(* Logix 5000 AddOnInstructionDefinition export AMCI_SV160E2_Axis_Follower_Circular; software revision 20.03 *)

ADD_ON_INSTRUCTION AMCI_SV160E2_Axis_Follower_Circular   (* revision 1.0, vendor AMCI, ExecuteEnableInFalse *)
// Revision note:
// 8/2019 Version 0 Initial release of SV160E2 Add On Instructions.
// 3/17/20 Version 13/17/20 Version 1 replaced the generic EDS file with a more complete V1.6 EDS file.  Also added a line of code to limit the minimum follower acceleration to -15999.
// Help:
// 2/2017: V0 is the initial release
// 7/2017: V1 added enable and error bits.
// 5/2019: V2 added unlatching the error bit when the rung goes false and the ability to select between normal (jog CCW) and continuous follower (jog CW)
VAR_OUTPUT
   EN : BOOL; {visible}
END_VAR
VAR_INPUT
   Status_Word_0 : INT; {required}
        .0   // set when moving CW
        .1   // set when moving CCW
        .3   // set when stopped
   Status_Word_1 : INT; {required}
        .15   // 0 when disabled 1 when enabled
   Follower_Position : REAL; {required}
   Follower_Velocity : REAL; {required}
   Follower_Acceleration : REAL; {required}
   Ramp_Acceleration : INT; {required}
   Deceleration : INT; {required}
   Conversion_Constant : REAL; {required}
   Position_Unwind : DINT; {required}
   Maximum_Move_Torque : INT;
END_VAR
VAR_IN_OUT
   AMCI_SV160E2_output_data : _000A:SV160E2_9125ACD4:O:0; {required}
END_VAR
VAR_OUTPUT
   Axis_Follower_occurring : BOOL; {visible}
   ER : BOOL; {visible}
END_VAR
VAR
   command_data_block : INT[10];
        [0]   // Command Bits MSW
        [1]   // Command Bits LSW
        [2]   // Upper Target Position
        [3]   // Lower Target Position
        [4]   // Upper Programmed Speed
        [5]   // Lower Programmed Speed
        [8]   // Unwind value when stopped, Maximum Move Torque when motion occurring
   axis_follower_position : DINT;
   axis_follower_velocity : DINT;
   axis_follower_acceleration : DINT; {access None}
END_VAR

ROUTINE EnableInFalse   (* ladder *)
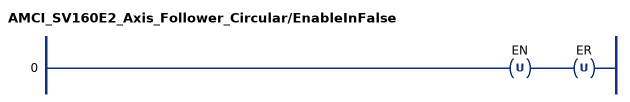
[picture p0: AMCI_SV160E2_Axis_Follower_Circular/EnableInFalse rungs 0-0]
   0: OTU(EN)OTU(ER);
END_ROUTINE

ROUTINE Logic   (* ladder *)
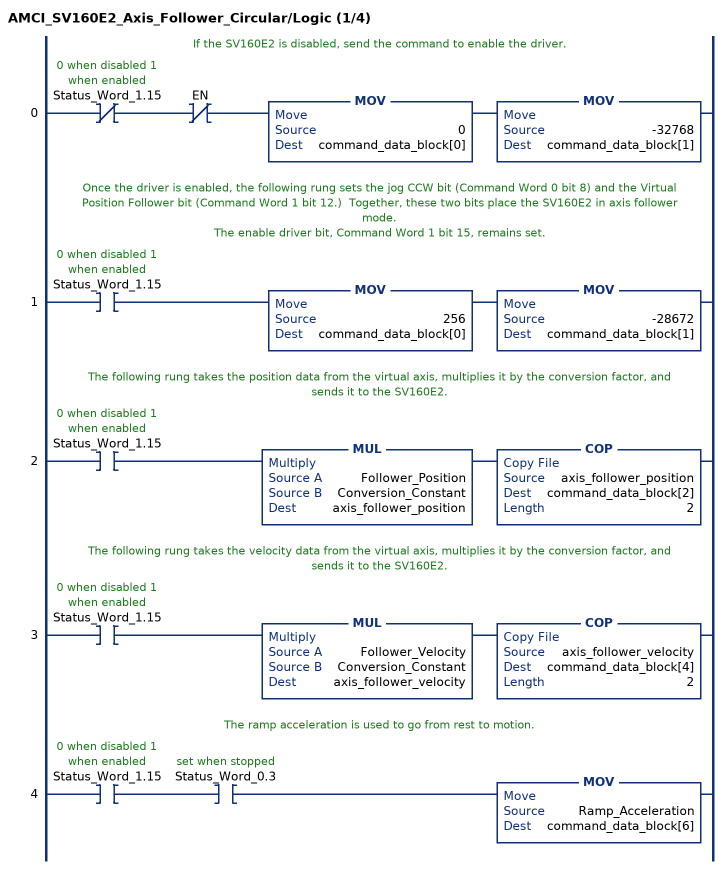
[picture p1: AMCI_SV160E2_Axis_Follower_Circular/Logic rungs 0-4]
   // If the SV160E2 is disabled, send the command to enable the driver.
   0: XIO(Status_Word_1.15)XIO(EN)MOV(0,command_data_block[0])MOV(-32768,command_data_block[1]);
   // Once the driver is enabled, the following rung sets the jog CCW bit (Command Word 0 bit 8) and the Virtual Position Follower bit (Command Word 1 bit 12.)  Together, these two bits place the SV160E2 in axis follower mode.
   // The enable driver bit, Command Word 1 bit 15, remains set.
   1: XIC(Status_Word_1.15)MOV(256,command_data_block[0])MOV(-28672,command_data_block[1]);
   // The following rung takes the position data from the virtual axis, multiplies it by the conversion factor, and sends it to the SV160E2.
   2: XIC(Status_Word_1.15)MUL(Follower_Position,Conversion_Constant,axis_follower_position)COP(axis_follower_position,command_data_block[2],2);
   // The following rung takes the velocity data from the virtual axis, multiplies it by the conversion factor, and sends it to the SV160E2.
   3: XIC(Status_Word_1.15)MUL(Follower_Velocity,Conversion_Constant,axis_follower_velocity)COP(axis_follower_velocity,command_data_block[4],2);
   // The ramp acceleration is used to go from rest to motion.
   4: XIC(Status_Word_1.15)XIC(Status_Word_0.3)MOV(Ramp_Acceleration,command_data_block[6]);
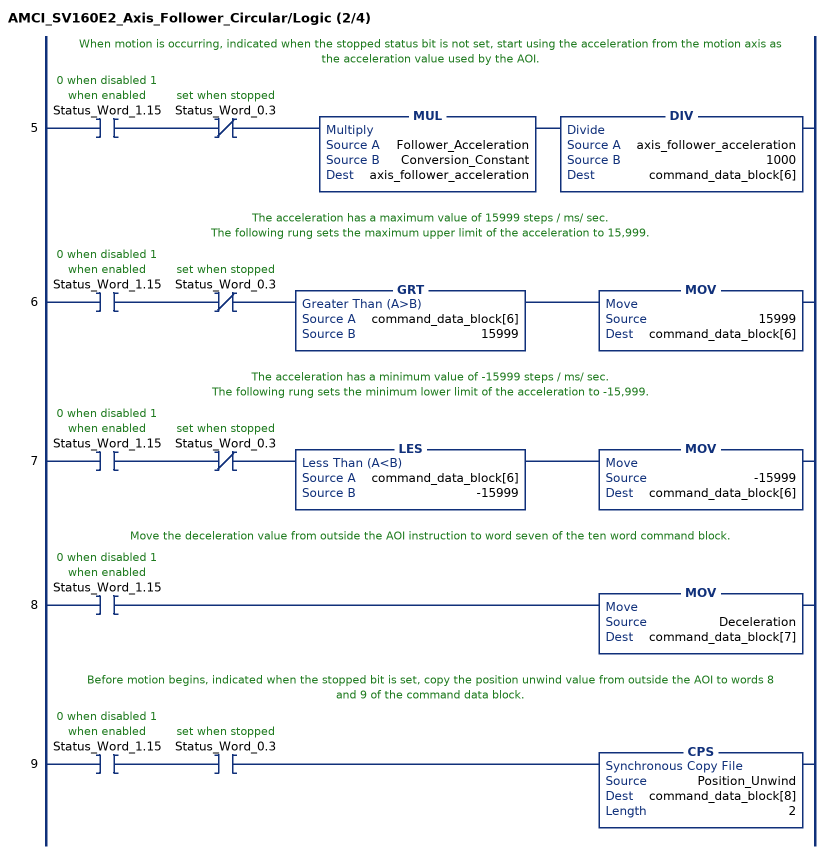
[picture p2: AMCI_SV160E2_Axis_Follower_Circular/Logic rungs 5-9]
   // When motion is occurring, indicated when the stopped status bit is not set, start using the acceleration from the motion axis as the acceleration value used by the AOI.
   5: XIC(Status_Word_1.15)XIO(Status_Word_0.3)MUL(Follower_Acceleration,Conversion_Constant,axis_follower_acceleration)DIV(axis_follower_acceleration,1000,command_data_block[6]);
   // The acceleration has a maximum value of 15999 steps / ms/ sec.
   // The following rung sets the maximum upper limit of the acceleration to 15,999.
   6: XIC(Status_Word_1.15)XIO(Status_Word_0.3)GRT(command_data_block[6],15999)MOV(15999,command_data_block[6]);
   // The acceleration has a minimum value of -15999 steps / ms/ sec.
   // The following rung sets the minimum lower limit of the acceleration to -15,999.
   7: XIC(Status_Word_1.15)XIO(Status_Word_0.3)LES(command_data_block[6],-15999)MOV(-15999,command_data_block[6]);
   // Move the deceleration value from outside the AOI instruction to word seven of the ten word command block.
   8: XIC(Status_Word_1.15)MOV(Deceleration,command_data_block[7]);
   // Before motion begins, indicated when the stopped bit is set, copy the position unwind value from outside the AOI to words 8 and 9 of the command data block.
   9: XIC(Status_Word_1.15)XIC(Status_Word_0.3)CPS(Position_Unwind,command_data_block[8],2);
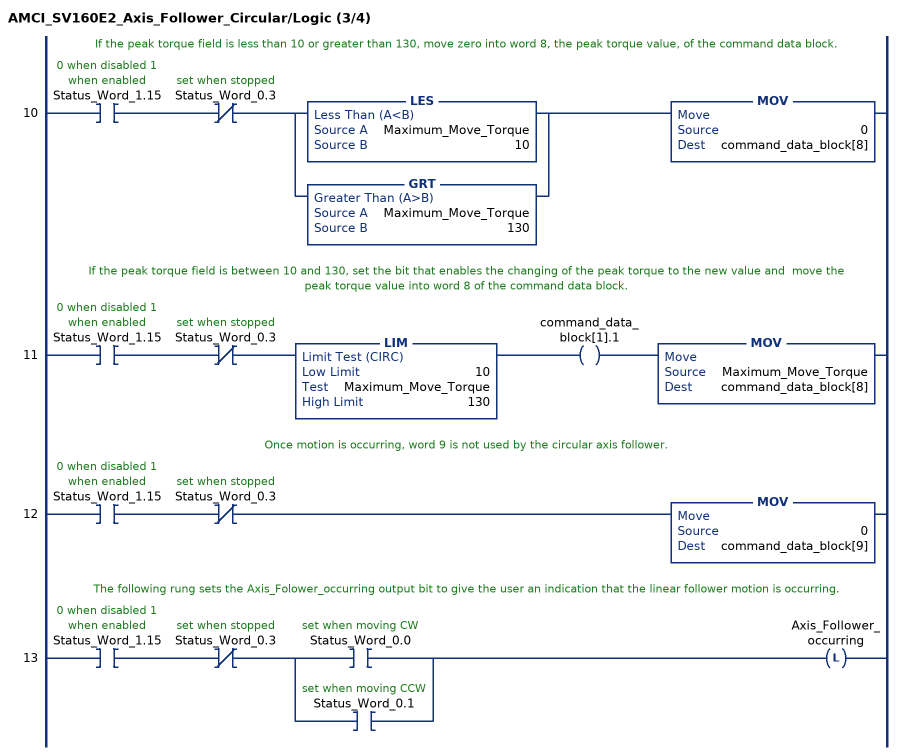
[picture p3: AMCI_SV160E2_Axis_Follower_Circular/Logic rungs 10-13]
   // If the peak torque field is less than 10 or greater than 130, move zero into word 8, the peak torque value, of the command data block.
   10: XIC(Status_Word_1.15)XIO(Status_Word_0.3)[LES(Maximum_Move_Torque,10) ,GRT(Maximum_Move_Torque,130) ]MOV(0,command_data_block[8]);
   // If the peak torque field is between 10 and 130, set the bit that enables the changing of the peak torque to the new value and  move the peak torque value into word 8 of the command data block.
   11: XIC(Status_Word_1.15)XIO(Status_Word_0.3)LIM(10,Maximum_Move_Torque,130)OTE(command_data_block[1].1)MOV(Maximum_Move_Torque,command_data_block[8]);
   // Once motion is occurring, word 9 is not used by the circular axis follower.
   12: XIC(Status_Word_1.15)XIO(Status_Word_0.3)MOV(0,command_data_block[9]);
   // The following rung sets the Axis_Folower_occurring output bit to give the user an indication that the linear follower motion is occurring.
   13: XIC(Status_Word_1.15)XIO(Status_Word_0.3)[XIC(Status_Word_0.0) ,XIC(Status_Word_0.1) ]OTL(Axis_Follower_occurring);
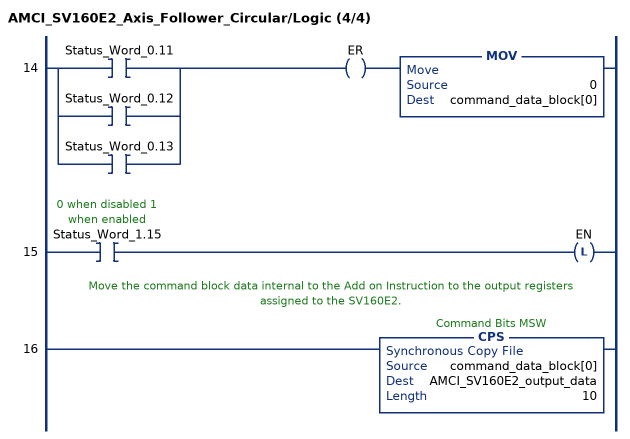
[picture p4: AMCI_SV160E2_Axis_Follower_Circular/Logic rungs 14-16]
   14: [XIC(Status_Word_0.11) ,XIC(Status_Word_0.12) ,XIC(Status_Word_0.13) ]OTE(ER)MOV(0,command_data_block[0]);
   15: XIC(Status_Word_1.15)OTL(EN);
   // Move the command block data internal to the Add on Instruction to the output registers assigned to the SV160E2.
   16: CPS(command_data_block[0],AMCI_SV160E2_output_data,10);
END_ROUTINE
END_ADD_ON_INSTRUCTION
